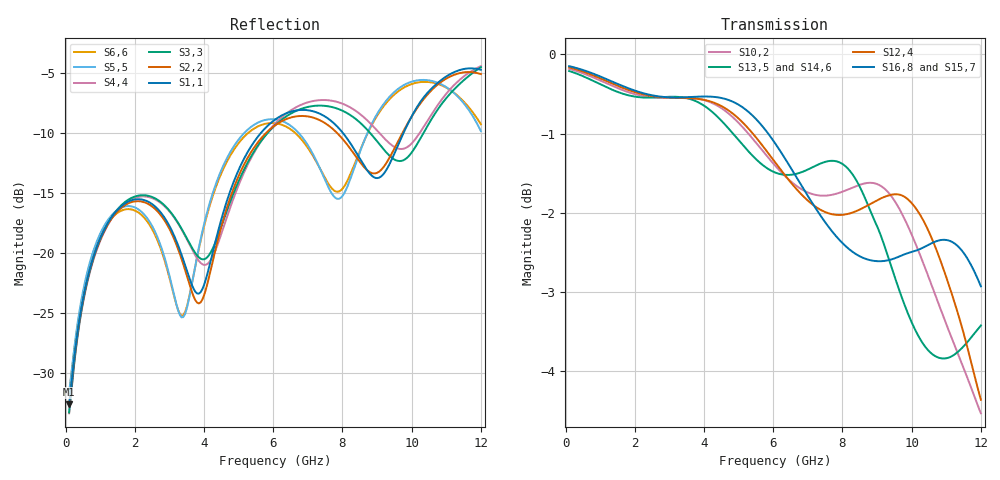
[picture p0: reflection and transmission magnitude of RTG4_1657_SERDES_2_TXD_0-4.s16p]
! RTG4 1657 S-parameter file
! Microsemi Corporation (c) 2019
!Initial ver: Jul 30, 2019
! Port::PIN_NAME::NET_NAME::S-parameter ports::PORT SIDE
! Port1:--:SERDES_2_TXD0_N_DIE::1::DIE
! Port2:--:SERDES_2_TXD0_P_DIE::2::DIE
! Port3:AT15:SERDES_2_TXD0_N_BGA::3::BGA
! Port4:AU15:SERDES_2_TXD0_P_BGA::4::BGA
! Port5:--:SERDES_2_TXD1_N_DIE::5::DIE
! Port6:--:SERDES_2_TXD1_P_DIE::6::DIE
! Port7:AT17:SERDES_2_TXD1_N_BGA::7::BGA
! Port8:AU17:SERDES_2_TXD1_P_BGA::8::BGA
! Port9:--:SERDES_2_TXD2_N_DIE::9::DIE
! Port10:--:SERDES_2_TXD2_P_DIE::10::DIE
! Port11:AV18:SERDES_2_TXD2_N_BGA::11::BGA
! Port12:AW18:SERDES_2_TXD2_P_BGA::12::BGA
! Port13:--:SERDES_2_TXD3_N_DIE::13::DIE
! Port14:--:SERDES_2_TXD3_P_DIE::14::DIE
! Port15:AT19:SERDES_2_TXD3_N_BGA::15::BGA
! Port16:AU19:SERDES_2_TXD3_P_BGA::16::BGA
!TouchstoneFormatFlag = 1
! GNDNET
! NETSLIST
! User Comments:
!  Touchstone file exported from HFSS 2018.2.0
!  File:  C:/Users/LSI_SIM_01/Desktop/Microsemi_190710/YBD197_150320_NETCHANGE_SERDES_2_TXD.aedt
!  Generated:  1:10:11  7 12, 2019
!  Design:  HFSSModel1
!  Project:  YBD197_150320_NETCHANGE_SERDES_2_TXD
!  Setup:  Setup1
!  Solution:  Sweep
! Terminal data exported
! Port[1] = SERDES_2_TXD0_N_DIE
! Port[2] = SERDES_2_TXD0_P_DIE
! Port[3] = SERDES_2_TXD1_N_DIE
! Port[4] = SERDES_2_TXD1_P_DIE
! Port[5] = SERDES_2_TXD2_N_DIE
! Port[6] = SERDES_2_TXD2_P_DIE
! Port[7] = SERDES_2_TXD3_N_DIE
! Port[8] = SERDES_2_TXD3_P_DIE
! Port[9] = SERDES_2_TXD0_N_BGA
! Port[10] = SERDES_2_TXD0_P_BGA
! Port[11] = SERDES_2_TXD1_N_BGA
! Port[12] = SERDES_2_TXD1_P_BGA
! Port[13] = SERDES_2_TXD2_N_BGA
! Port[14] = SERDES_2_TXD2_P_BGA
! Port[15] = SERDES_2_TXD3_N_BGA
! Port[16] = SERDES_2_TXD3_P_BGA
# GHZ S DB R 50.000000
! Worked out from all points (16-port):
!   239 points, 100 MHz to 12 GHz, reference 50 ohm
!   strongest paths, dB at 100 MHz, 3.05 GHz, 6.05 GHz, 9.05 GHz, 12 GHz:
!     S16,8: -0.1, -0.5, -1.1, -2.6, -2.9
!     S15,7: -0.1, -0.6, -1.1, -2.5, -2.9
!     S12,4: -0.2, -0.5, -1.4, -1.8, -4.4
!     S13,5: -0.2, -0.5, -1.5, -2.2, -3.4
!     S14,6: -0.2, -0.5, -1.5, -2.1, -3.3
!     S10,2: -0.2, -0.5, -1.4, -1.6, -4.5
!   lowest |S11| = -32.6 dB at 100 MHz (marker M1), VSWR 1.05, Z = 52 - j1.34 ohm
!   |S11| at or under -10 dB: start of sweep to 5.643 GHz; 8.011 GHz to 9.765 GHz (1.755 GHz wide, 19.7 % of centre)
